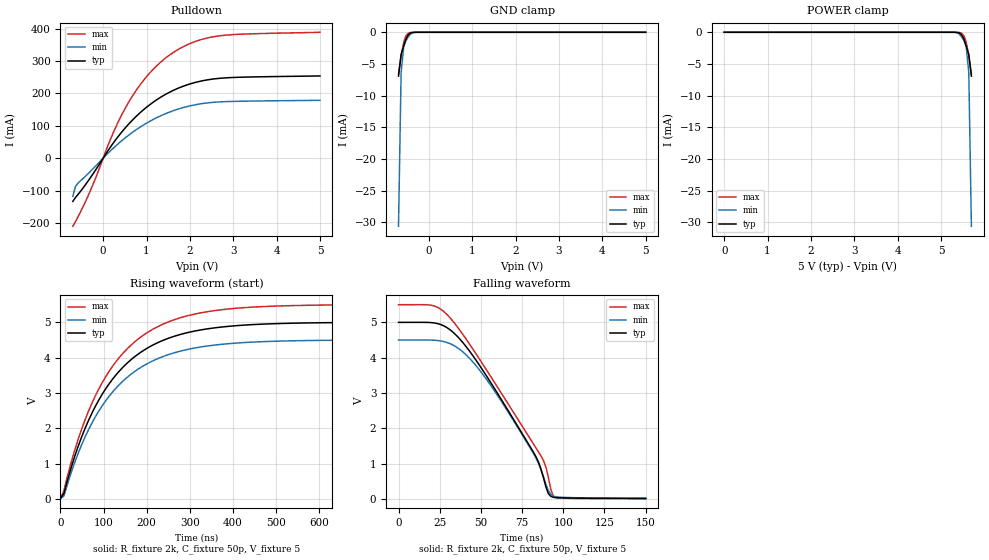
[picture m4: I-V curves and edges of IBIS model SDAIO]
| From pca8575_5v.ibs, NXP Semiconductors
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[Model]   SDAIO
Model_type I/O_open_drain
Enable Active-Low
Vinh=3.5
Vinl=1.5
Vref=5
Vmeas=2.5
Rref=2k
Cref=50p
C_comp   8p   7.8p   8.2p
[Temperature Range] 27   85   -40
[Voltage Range]   5   4.5   5.5
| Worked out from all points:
|   slope of the pulldown table from 0 to 0.75 V, typ, clamps not added: 5.87 ohm
|   GND clamp passes 1 mA (typ) near -0.52 V on its own axis
|   falling waveform, R_fixture 2k, C_fixture 50p, V_fixture 5: 20-80 % time 39.3ns typ, 35.8ns min, 44.9ns max; typ from 5 V to 0.016 V
|   rising waveform, R_fixture 2k, C_fixture 50p, V_fixture 5: 20-80 % time 142ns typ, 142ns min, 141ns max; typ from 0.012 V to 5 V
[Pulldown]
-700mV    -133.4mA   -118.1mA   -210.3mA
-640mV    -121.8mA   -87.63mA   -196.3mA
-580mV    -111.9mA   -77.16mA   -181.2mA
-240mV    -49.58mA   -33.19mA   -82.87mA
220mV     44.25mA    29.24mA    74.72mA
510mV     93.65mA    62.95mA    154.5mA
740mV     126.4mA    85.93mA    205.2mA
970mV     154mA      105.8mA    246.8mA
1.43V     196.4mA    137mA      308.2mA
1.95V     227mA      159.9mA    350.9mA
2.58V     245.2mA    172.9mA    375.8mA
5V        254mA      178.7mA    388.8mA
[GND Clamp]
-700mV    -6.935mA   -30.66mA   -6.593mA
-640mV    -3.526mA   -6.329mA   -3.662mA
-580mV    -2.155mA   -2.263mA   -1.567mA
-530mV    -1.094mA   -1.347mA   -591uA
-470mV    -356.7uA   -681.6uA   -111.6uA
-410mV    -74.12uA   -204.6uA   -11.6uA
-350mV    -9.861uA   -39.84uA   -825nA
-240mV    -132.3nA   -884.3nA   -4.564nA
5V        281.2pA    510.1pA    260.2pA
[POWER Clamp]
0V        281.2pA    510.1pA    260.2pA
5.24V     -132.3nA   -884.3nA   -4.564nA
5.35V     -9.861uA   -39.84uA   -825nA
5.41V     -74.12uA   -204.6uA   -11.6uA
5.47V     -356.7uA   -681.6uA   -111.6uA
5.53V     -1.094mA   -1.347mA   -591uA
5.58V     -2.155mA   -2.263mA   -1.567mA
5.64V     -3.526mA   -6.329mA   -3.662mA
5.7V      -6.935mA   -30.66mA   -6.593mA
[Falling Waveform]
R_fixture=2k
C_fixture=50p
V_fixture=5
V_fixture_min=4.5
V_fixture_max=5.5
0s        5V         4.5V       5.5V
24.24ns   4.959V     4.484V     5.413V
33.33ns   4.711V     4.351V     5.016V
42.42ns   4.23V      4.016V     4.432V
66.67ns   2.494V     2.453V     2.683V
83.33ns   1.208V     1.168V     1.451V
87.88ns   618mV      642.1mV    1.101V
90.91ns   154.7mV    243.6mV    622mV
93.94ns   49.98mV    85.95mV    78.44mV
150ns     15.63mV    22.5mV     9.732mV
[Rising Waveform]
R_fixture=2k
C_fixture=50p
V_fixture=5
V_fixture_min=4.5
V_fixture_max=5.5
0s        11.69mV    16.13mV    7.463mV
8.081ns   158mV      81.67mV    237.9mV
24.24ns   863mV      721.2mV    1.006V
48.48ns   1.734V     1.515V     1.954V
88.89ns   2.799V     2.486V     3.113V
145.5ns   3.735V     3.341V     4.129V
210.1ns   4.328V     3.884V     4.773V
282.8ns   4.671V     4.197V     5.144V
387.9ns   4.882V     4.392V     5.373V
800ns     4.998V     4.498V     5.498V
[Ramp]
R_load=2k
dV/dt_r   2.993E+0/3.314E-9   2.989E+0/3.629E-9   2.996E+0/2.988E-9
dV/dt_f   2.991E+0/3.908E-8   2.985E+0/3.903E-8   2.995E+0/4.071E-8
|[End   SDAIO
